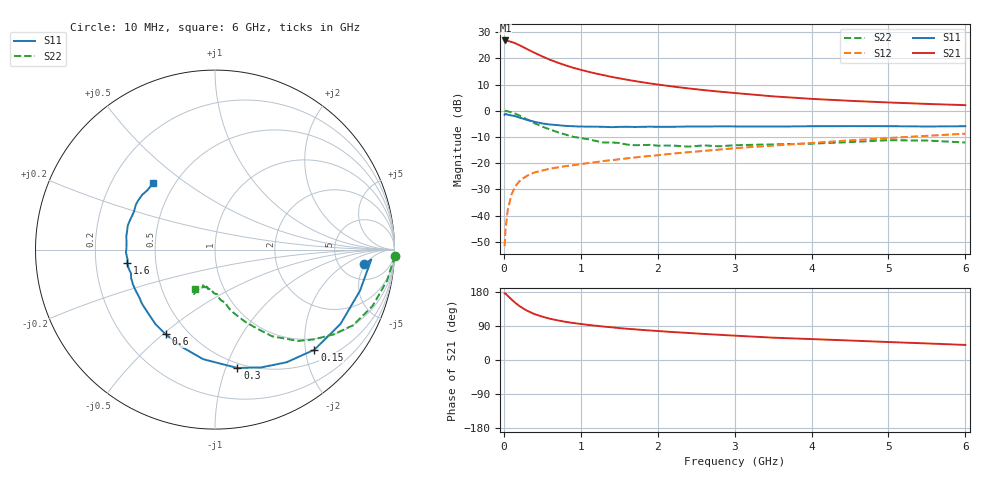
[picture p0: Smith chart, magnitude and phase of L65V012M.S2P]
!  INFINEON TECHNOLOGIES Small Signal Semiconductors
! BFR380L3 , Si-NPN RF-Transistor in TSLP-3-1
!  Vce=5 V,  Ic=12.5 mA
! Common Emitter S-Parameters:  07. March 2005
#  GHz  S  MA  R  50
! f  S11  S21  S12  S22
! GHz  Mag  Ang  Mag  Ang  Mag  Ang  Mag  Ang
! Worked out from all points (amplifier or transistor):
!   36 points, 10 MHz to 6 GHz, reference 50 ohm
!   highest |S21| = 26.8 dB at 20 MHz (marker M1)
!   |S21| within 3 dB of that: start of sweep to 282.3 MHz
!   unconditionally stable (mu >= 1): 2.387 GHz to 4.669 GHz
!   at 250 MHz: K = 0.24, MSG = 25.1 dB, |S12| = -25.8 dB
!   at 1.4 GHz: K = 0.86, MSG = 15.9 dB, |S12| = -18.9 dB
!   at 6 GHz: K = 0.96, MSG = 5.5 dB, |S12| = -8.8 dB
!   S11 on the Smith chart (normalised r, x): 10 MHz: 8.73, -4.67; 150 MHz: 0.75, -2.19; 300 MHz: 0.46, -1.10; 600 MHz: 0.38, -0.51; 1.6 GHz: 0.34, -0.07; 6 GHz: 0.38, +0.38
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0.01  0.8367 -5.5  21.97 175.9  0.0026 83.2  1.005 -2.0
0.02  0.8727 -3.6  21.98 175.9  0.005 84.8  0.9928 -4.2
0.05  0.8398 -15.8  21.56 169.4  0.0127 83.0  0.9745 -10.1
0.1  0.8129 -30.6  20.57 159.8  0.0253 76.3  0.9325 -19.7
0.15  0.786 -45.2  19.41 150.7  0.0361 68.8  0.8775 -28.7
0.2  0.7437 -57.6  17.93 142.8  0.0447 64.0  0.813 -35.5
0.25  0.7047 -68.7  16.49 136.3  0.0512 59.5  0.7432 -42.3
0.3  0.6711 -79.3  15.07 130.3  0.0573 56.2  0.6869 -47.8
0.4  0.6144 -96.1  12.75 121.0  0.0665 51.6  0.5775 -56.7
0.5  0.5725 -109.0  10.89 114.4  0.0722 50.0  0.4978 -62.0
0.6  0.5461 -120.3  9.404 108.8  0.0784 48.5  0.4384 -67.1
0.7  0.5317 -128.5  8.291 104.6  0.0829 48.7  0.3894 -71.3
0.8  0.5141 -136.3  7.386 100.8  0.0875 48.5  0.352 -75.4
1.1  0.4974 -152.8  5.549 92.5  0.1003 50.5  0.2863 -82.9
1.4  0.4867 -164.1  4.435 86.3  0.1139 52.6  0.2483 -88.6
1.6  0.4949 -171.2  3.915 82.5  0.1235 53.8  0.226 -95.2
2.2  0.4942 175.5  2.899 73.7  0.1522 57.0  0.2164 -100.9
2.8  0.504 164.7  2.319 66.5  0.1815 59.2  0.2096 -108.5
3.5  0.4986 154.8  1.884 58.9  0.2164 59.2  0.2285 -111.3
4.5  0.5082 147.4  1.548 51.4  0.2717 60.0  0.2522 -113.9
5.5  0.5012 138.5  1.351 43.7  0.3322 58.3  0.2697 -115.8
6  0.5067 132.8  1.28 39.8  0.3649 56.8  0.248 -116.8
